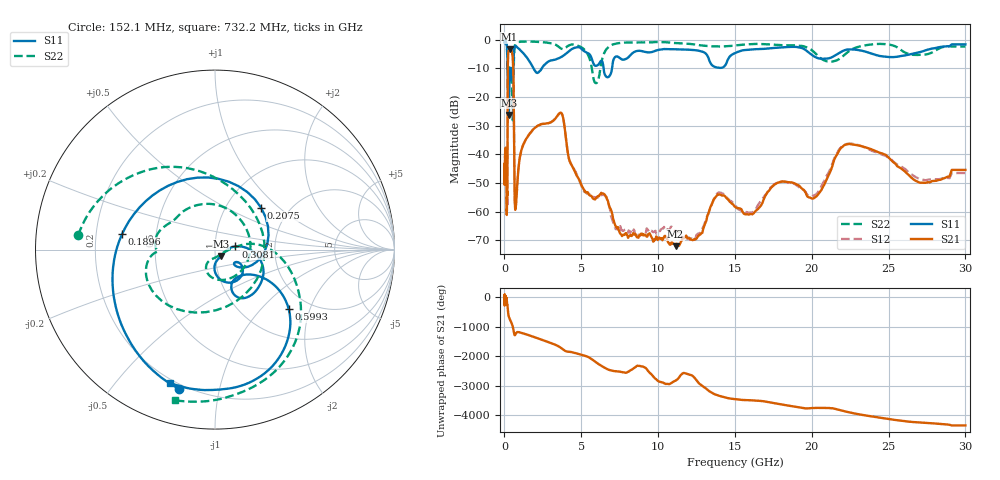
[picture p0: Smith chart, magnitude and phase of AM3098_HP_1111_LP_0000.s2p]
! Date/Time: Thu, Feb 28, 2019 8:47 AM
! Network Analyzer: Agilent Technologies E8364B Rev: A.07.50.67
! Sweep from 0.010 to 30.000 GHz, 1601 Points, Sweep Type: LOG
! Power Supply: 5.022 V, 0.002 A
# Hz S DB R 50
!freq MagS11 AngS11 MagS21 AngS21 MagS12 AngS12 MagS22 AngS22
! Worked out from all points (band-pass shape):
!   1601 points, 10 MHz to 30 GHz, reference 50 ohm
!   highest |S21| = -3.30 dB at 335.4 MHz (marker M1); lowest = -72.1 dB at 11.14 GHz (marker M2)
!   |S21| within 3 dB of the highest: 228 MHz to 539.3 MHz (311.2 MHz wide, 81.1 % of centre)
!   lowest |S11| = -26.2 dB at 288.7 MHz (marker M3), VSWR 1.10, Z = 53.3 - j3.82 ohm
!   |S11| at or under -10 dB: 210 MHz to 381.4 MHz (171.4 MHz wide, 58 % of centre); 1.889 GHz to 2.424 GHz (535.1 MHz wide, 24.8 % of centre); 6.454 GHz to 7.001 GHz (547 MHz wide, 8.13 % of centre)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
!   |S22| runs from -28.1 to -0.4 dB; largest |S21 - S12| = 0.012
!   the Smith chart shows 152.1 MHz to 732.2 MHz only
!   S11 on the Smith chart (normalised r, x): 152.1 MHz: 0.18, -0.76; 189.6 MHz: 0.31, +0.07; 207.5 MHz: 1.45, +0.77; 308.1 MHz: 1.25, +0.04; 599.3 MHz: 1.57, -1.45; 732.2 MHz: 0.18, -0.70
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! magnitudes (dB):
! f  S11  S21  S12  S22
! 10 MHz  -0.3  -47.6  -43.6  -0.5
! 38.04 MHz  -0.2  -40.8  -41.1  -0.5
! 108.3 MHz  -1.0  -40.6  -40.6  -1.2
! 144.7 MHz  -1.6  -57.6  -54.8  -2.0
! 152.1 MHz  -1.9  -61.2  -57.8  -2.3
! 189.6 MHz  -5.6  -51.4  -51.0  -9.6
! 207.5 MHz  -9.2  -20.1  -20.2  -8.4
! 288.7 MHz  -26.2  -3.5  -3.4  -10.5
! 308.1 MHz  -18.8  -3.4  -3.3  -11.0
! 335.4 MHz  -12.3  -3.3  -3.3  -11.2
! 550.5 MHz  -12.6  -7.2  -7.1  -27.0
! 599.3 MHz  -5.5  -18.5  -18.4  -10.2
! 665.8 MHz  -2.2  -55.6  -54.8  -2.3
! 732.2 MHz  -2.1  -58.3  -58.3  -1.2
! 2.084 GHz  -11.5  -30.3  -30.4  -0.7
! 3.686 GHz  -6.1  -25.5  -25.5  -3.1
! 5.959 GHz  -9.1  -55.2  -55.1  -15.1
! 7.926 GHz  -6.6  -67.5  -66.8  -1.0
! 11.14 GHz  -3.3  -72.1  -66.6  -1.1
! 20 GHz  -5.3  -55.4  -54.7  -3.6
! 22.56 GHz  -3.4  -36.5  -36.2  -3.5
! 30 GHz  -1.6  -45.4  -46.5  -2.4
